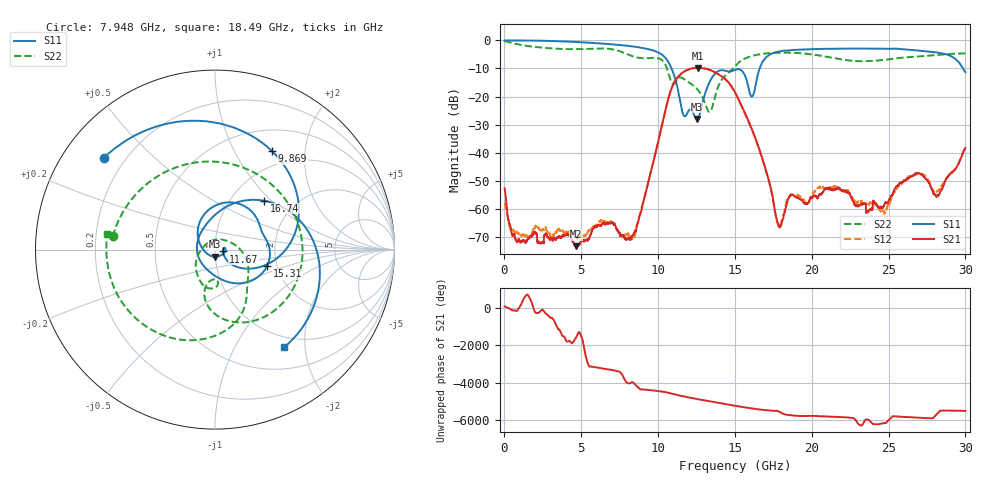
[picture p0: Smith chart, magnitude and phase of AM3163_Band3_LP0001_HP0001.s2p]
!Agilent Technologies,E8364B,MY43040894,A.07.50.67
!Agilent E8364B: A.07.50.67
!Date: Thursday, August 20, 2020 11:04:20
!Correction: S11(Full 2 Port(1,2))
!S21(Full 2 Port(1,2))
!S12(Full 2 Port(1,2))
!S22(Full 2 Port(1,2))
!S2P File: Measurements: S11, S21, S12, S22:
# Hz S  dB  R 50
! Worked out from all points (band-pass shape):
!   3201 points, 10 MHz to 30 GHz, reference 50 ohm
!   highest |S21| = -9.78 dB at 12.62 GHz (marker M1); lowest = -73.2 dB at 4.64 GHz (marker M2)
!   |S21| within 3 dB of the highest: 11.33 GHz to 14.14 GHz (2.811 GHz wide, 22.1 % of centre)
!   lowest |S11| = -27.9 dB at 12.52 GHz (marker M3), VSWR 1.08, Z = 49.8 - j4 ohm
!   |S11| at or under -10 dB: 10.87 GHz to 16.61 GHz (5.733 GHz wide, 41.7 % of centre); 29.83 GHz to end of sweep
!   |S22| runs from -25.5 to -0.3 dB; largest |S21 - S12| = 0.0044
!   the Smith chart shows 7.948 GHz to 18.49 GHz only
!   S11 on the Smith chart (normalised r, x): 7.948 GHz: 0.12, +0.35; 9.869 GHz: 0.78, +1.43; 11.67 GHz: 1.09, -0.02; 15.31 GHz: 1.77, -0.36; 16.74 GHz: 1.41, +0.90; 18.49 GHz: 0.82, -1.61
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1e7  -0.03 -1.9  -52.70 64.4  -57.87 -42.6  -0.32 -7.0
9.471875e8  -0.05 -26.0  -70.67 -8.4  -68.82 80.5  -1.47 -84.5
2.174903e9  -0.12 -59.7  -72.11 67.5  -66.03 8.1  -2.46 -166.0
4.639706e9  -0.57 -125.6  -73.23 168.0  -69.70 -8.5  -3.12 63.2
5.014581e9  -0.68 -135.5  -71.20 -121.7  -70.01 -101.0  -3.09 42.1
6.795238e9  -1.31 175.7  -65.01 -64.8  -64.75 -71.6  -3.01 -79.0
7.947978e9  -1.90 140.4  -70.97 -35.3  -68.82 -59.1  -4.81 172.7
8.782075e9  -2.50 110.7  -62.83 -16.1  -62.43 -48.2  -6.25 82.8
9.869212e9  -3.96 59.9  -39.20 -117.7  -39.32 -118.8  -6.25 -26.0
1.000979e10  -4.30 51.5  -35.94 -132.0  -36.07 -132.9  -6.38 -39.9
1.166861e10  -26.73 -12.9  -11.17 -62.4  -11.27 -62.3  -13.67 -109.1
1.252145e10  -27.94 -90.3  -9.79 160.0  -9.84 160.4  -17.20 -141.2
1.261517e10  -27.56 -120.4  -9.78 146.0  -9.82 146.3  -17.80 -145.8
1.5005e10  -10.49 5.4  -18.47 158.8  -18.68 159.0  -9.24 -60.5
1.531427e10  -10.34 -17.6  -21.85 115.6  -22.06 116.1  -7.60 -73.4
1.67388e10  -8.28 45.0  -41.19 -52.8  -41.56 -50.4  -4.85 -130.0
1.784468e10  -3.99 -28.7  -66.25 -147.7  -65.75 35.1  -4.39 -166.8
1.849134e10  -3.52 -54.7  -56.22 24.5  -55.93 26.8  -4.36 171.9
2.000958e10  -3.12 -99.6  -55.94 -19.4  -55.25 -28.4  -4.98 117.8
2.24369e10  -2.93 -156.4  -54.28 -114.0  -54.16 -112.5  -7.16 9.5
2.500479e10  -3.01 144.5  -56.95 110.0  -58.58 -73.0  -6.77 -104.1
3e10  -11.30 -20.7  -38.26 -118.0  -38.24 -113.7  -4.65 99.5
